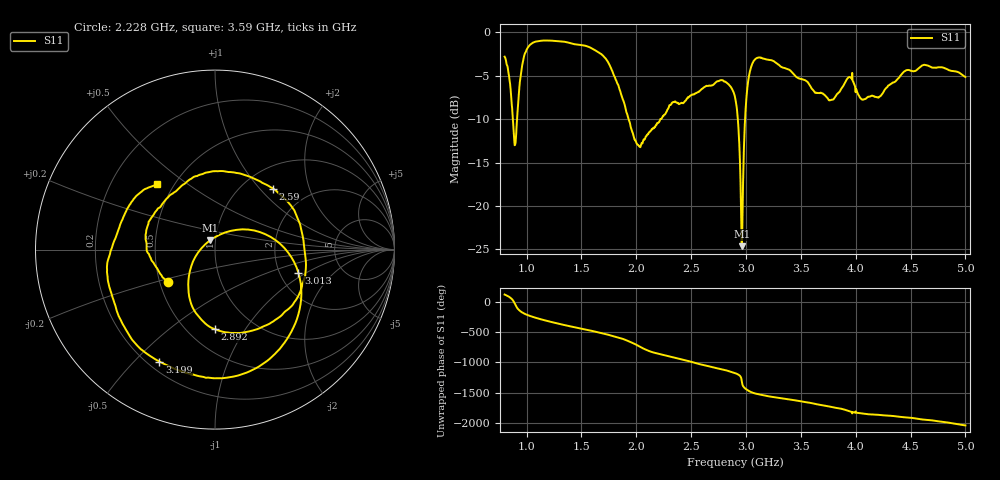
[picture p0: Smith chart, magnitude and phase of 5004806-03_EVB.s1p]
#  HZ  S  RI  R  50.00
! Rohde & Schwarz ZVA/B
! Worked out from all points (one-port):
!   1601 points, 800 MHz to 5 GHz, reference 50 ohm
!   lowest |S11| = -24.6 dB at 2.963 GHz (marker M1), VSWR 1.12, Z = 47 + j4.83 ohm
!   |S11| at or under -10 dB: 875.2 MHz to 913.2 MHz (38.02 MHz wide, 4.25 % of centre); 1.93 GHz to 2.219 GHz (288.8 MHz wide, 13.9 % of centre); 2.926 GHz to 2.992 GHz (65.8 MHz wide, 2.22 % of centre)
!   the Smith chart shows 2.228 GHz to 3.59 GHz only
!   S11 on the Smith chart (normalised r, x): 2.228 GHz: 0.55, -0.22; 2.59 GHz: 1.36, +1.19; 2.892 GHz: 0.67, -0.74; 3.013 GHz: 2.53, -0.84; 3.199 GHz: 0.24, -0.59; 3.59 GHz: 0.41, +0.39
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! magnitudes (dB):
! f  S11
! 800 MHz  -2.8
! 836.8 MHz  -4.8
! 894.5 MHz  -13.0
! 954.9 MHz  -4.2
! 1.002 GHz  -2.0
! 1.325 GHz  -1.0
! 1.682 GHz  -2.5
! 1.85 GHz  -6.6
! 2.021 GHz  -13.0
! 2.228 GHz  -10.0
! 2.375 GHz  -8.1
! 2.59 GHz  -6.6
! 2.779 GHz  -5.5
! 2.892 GHz  -7.1
! 2.9 GHz  -7.4
! 2.924 GHz  -9.6
! 2.95 GHz  -17.1
! 2.963 GHz  -24.6
! 3.013 GHz  -6.3
! 3.073 GHz  -3.2
! 3.199 GHz  -3.1
! 3.425 GHz  -4.7
! 3.59 GHz  -6.3
! 3.777 GHz  -7.8
! 3.95 GHz  -5.2
! 4.073 GHz  -7.7
! 4.475 GHz  -4.3
! 5 GHz  -5.1
